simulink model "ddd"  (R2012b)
settings: Solver=ode45  StartTime=0.0  StopTime=1  RelTol=1e-3
undefined symbols (not defined in the file): d, Gg, Jgls, Jt, k, tavb, tavg
libraries: fuzblock x1, re_lib x1

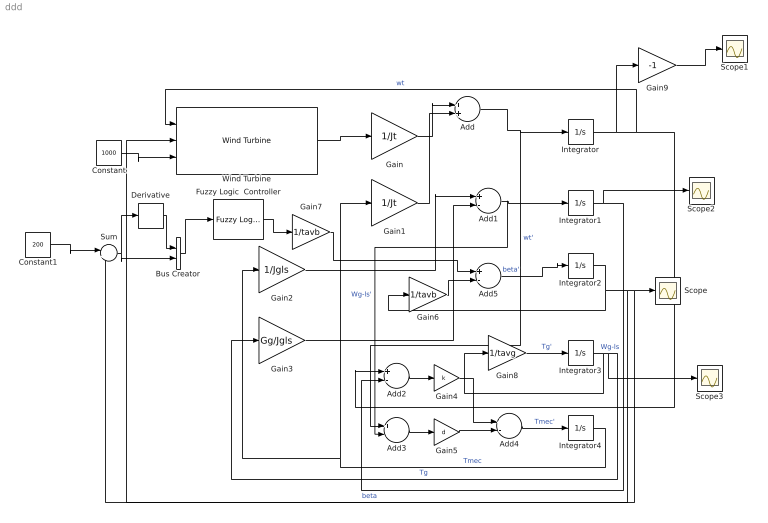
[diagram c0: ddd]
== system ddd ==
  Add : Sum
  Add{1..5} (5 alike) : Sum  Inputs=+-
  Bus Creator : BusCreator  Inputs=2
  Constant : Constant  Value=1000
  Constant1 : Constant  Value=200
  Derivative : Derivative
  Fuzzy Logic  Controller : fuzblock/Fuzzy Logic  Controller  fis=f
  Gain : Gain  Gain=1/Jt
  Gain1 : Gain  Gain=1/Jt
  Gain2 : Gain  Gain=1/Jgls
  Gain3 : Gain  Gain=Gg/Jgls
  Gain4 : Gain  Gain=k
  Gain5 : Gain  Gain=d
  Gain6 : Gain  Gain=1/tavb
  Gain7 : Gain  Gain=1/tavb
  Gain8 : Gain  Gain=1/tavg
  Gain9 : Gain  Gain=-1
  Integrator{,1..4} (5 alike) : Integrator
  Scope{,1..3} (4 alike) : Scope
  Sum : Sum  Inputs=|+-
  Wind Turbine : re_lib/Wind Generation/Wind Turbine  Pnom=.9e6  Pelec_base=1.5e6/0.9  wind_base=12  P_wind_base=0.73  speed_nom=1.2  pitch_angle=0  DisplayTurbChar=off  c1_c6="[0.51763          116          0.4            5           21     0.006795]"  cp_nom=0.48  lambda_nom=8.1
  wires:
  Integrator1/1 -> Scope2/1, Add2/2  "Wg-ls"
  Add1/1 -> Integrator1/1, Add3/2  "Wg-ls'"
  Integrator4/1 -> Gain2/1, Gain1/1  "Tmec"
  Add4/1 -> Integrator4/1  "Tmec'"
  Integrator3/1 -> Gain8/1, Scope3/1, Gain3/1  "Tg"
  Gain8/1 -> Integrator3/1  "Tg'"
  Integrator2/1 -> Wind Turbine/2, Sum/2, Scope/1, Gain6/1  "beta"
  Add5/1 -> Integrator2/1  "beta'"
  Integrator/1 -> Gain9/1, Wind Turbine/1, Add2/1  "wt"
  Add/1 -> Integrator/1, Add3/1  "wt'"
  Wind Turbine/1 -> Gain/1
  Gain/1 -> Add/1
  Gain1/1 -> Add/2
  Gain2/1 -> Add1/1
  Gain3/1 -> Add1/2
  Add3/1 -> Gain5/1
  Gain5/1 -> Add4/2
  Add2/1 -> Gain4/1
  Gain4/1 -> Add4/1
  Gain6/1 -> Add5/2
  Gain7/1 -> Add5/1
  Constant/1 -> Wind Turbine/3
  Gain9/1 -> Scope1/1
  Fuzzy Logic  Controller/1 -> Gain7/1
  Constant1/1 -> Sum/1
  Bus Creator/1 -> Fuzzy Logic  Controller/1
  Derivative/1 -> Bus Creator/1
  Sum/1 -> Derivative/1, Bus Creator/2
